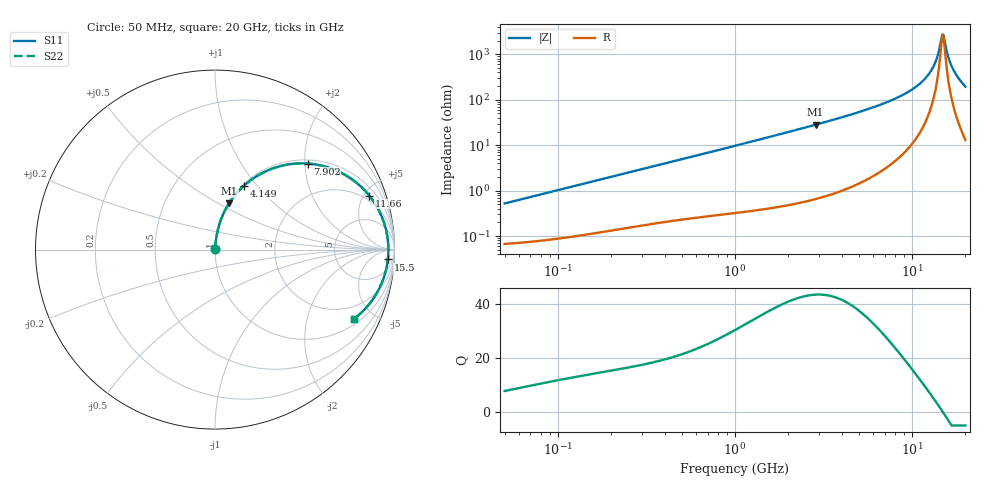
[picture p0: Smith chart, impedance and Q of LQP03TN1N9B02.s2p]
!Murata Part Number: LQP03TN1N9B02
!These Parameters are Measured in Series Mode Connection
!  o--[Z]--o
!Port1  Port2
!  o-------o
!Freq. Start=50[MHz] Stop=20[GHz], 401[Steps]
# Hz S RI R 50
!Freq.(Hz) S11(Real) S11(Imag) S21(Real) S21(Imag) S12(Real) S12(Imag) S22(Real) S22(Imag)
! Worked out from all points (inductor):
!   401 points, 50 MHz to 20 GHz, reference 50 ohm
!   read as one part in series: L = 1.65 nH near 51.52 MHz
!   highest Q = 43.4 at 2.853 GHz (marker M1), where L = 1.58 nH
!   self-resonance near 14.82 GHz
!   S11 on the Smith chart (normalised r, x): 50 MHz: 1.00, +0.01; 4.149 GHz: 1.02, +0.86; 7.902 GHz: 1.09, +2.06; 11.66 GHz: 1.55, +5.47; 15.5 GHz: 16, -25; 20 GHz: 1.26, -3.88
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5e7  0.000699 0.00519  0.9993 -0.00519  0.9993 -0.00519  0.000699 0.00519
1.364002e8  0.00123 0.0139  0.9988 -0.0139  0.9988 -0.0139  0.00123 0.0139
3.721004e8  0.0033 0.0366  0.9967 -0.0366  0.9967 -0.0366  0.0033 0.0366
1e9  0.0124 0.0955  0.9876 -0.0955  0.9876 -0.0955  0.0124 0.0955
2.728004e9  0.0729 0.2486  0.9271 -0.2486  0.9271 -0.2486  0.0729 0.2486
2.853386e9  0.0793 0.2589  0.9207 -0.2589  0.9207 -0.2589  0.0793 0.2589
4.149438e9  0.1611 0.3556  0.8389 -0.3556  0.8389 -0.3556  0.1611 0.3556
5.598765e9  0.2821 0.4359  0.7179 -0.4359  0.7179 -0.4359  0.2821 0.4359
7.442007e9  0.4669 0.4802  0.5331 -0.4802  0.5331 -0.4802  0.4669 0.4802
7.901521e9  0.5155 0.4795  0.4845 -0.4795  0.4845 -0.4795  0.5155 0.4795
9.892087e9  0.7174 0.4204  0.2826 -0.4204  0.2826 -0.4204  0.7174 0.4204
1.166392e10  0.8599 0.3004  0.1401 -0.3004  0.1401 -0.3004  0.8599 0.3004
1.257102e10  0.9112 0.222  0.0888 -0.222  0.0888 -0.222  0.9112 0.222
1.334722e10  0.9417 0.1498  0.0583 -0.1498  0.0583 -0.1498  0.9417 0.1498
1.460232e10  0.965 0.0296  0.035 -0.0296  0.035 -0.0296  0.965 0.0296
1.482269e10  0.9659 0.00859  0.0341 -0.00859  0.0341 -0.00859  0.9659 0.00859
1.504638e10  0.9658 -0.0125  0.0342 0.0125  0.0342 0.0125  0.9658 -0.0125
1.550395e10  0.9629 -0.0551  0.0371 0.0551  0.0371 0.0551  0.9629 -0.0551
1.621653e10  0.9513 -0.1189  0.0487 0.1189  0.0487 0.1189  0.9513 -0.1189
1.696185e10  0.9308 -0.1818  0.0692 0.1818  0.0692 0.1818  0.9308 -0.1818
1.828096e10  0.8764 -0.2811  0.1236 0.2811  0.1236 0.2811  0.8764 -0.2811
2e10  0.7757 -0.3849  0.2243 0.3849  0.2243 0.3849  0.7757 -0.3849
